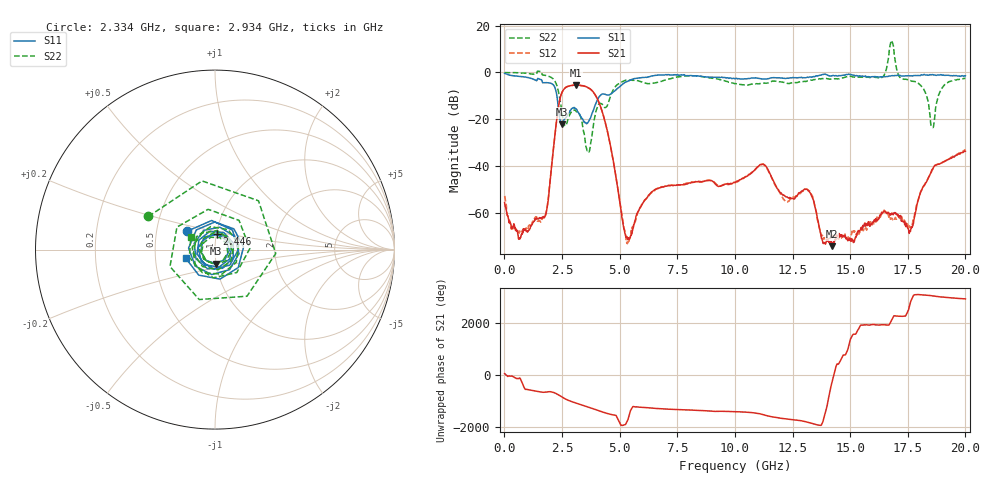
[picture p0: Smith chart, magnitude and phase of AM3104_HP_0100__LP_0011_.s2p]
!Created with skrf (http://scikit-rf.org).
# Hz S RI R 50.0
!freq ReS11 ImS11 ReS21 ImS21 ReS12 ImS12 ReS22 ImS22
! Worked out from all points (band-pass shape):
!   1601 points, 10 MHz to 20 GHz, reference 50 ohm
!   highest |S21| = -5.36 dB at 3.108 GHz (marker M1); lowest = -74.2 dB at 14.2 GHz (marker M2)
!   |S21| within 3 dB of the highest: 2.506 GHz to 3.857 GHz (1.351 GHz wide, 42.5 % of centre)
!   lowest |S11| = -22.2 dB at 2.496 GHz (marker M3), VSWR 1.17, Z = 49.7 - j7.77 ohm
!   |S11| at or under -10 dB: 2.279 GHz to 4.146 GHz (1.867 GHz wide, 58.1 % of centre)
!   |S22| runs from -34.0 to 13.7 dB; largest |S21 - S12| = 0.03
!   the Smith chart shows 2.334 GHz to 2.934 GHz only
!   S11 on the Smith chart (normalised r, x): 2.334 GHz: 0.72, +0.15; 2.446 GHz: 1.00, +0.17; 2.934 GHz: 0.72, -0.07
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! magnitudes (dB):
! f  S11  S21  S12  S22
! 10 MHz  -0.4  -55.6  -52.7  0.0
! 672.2 MHz  -1.7  -70.8  -67.7  -0.2
! 1.684 GHz  -4.4  -61.6  -62.0  -1.1
! 2.334 GHz  -14.7  -15.4  -15.5  -7.7
! 2.446 GHz  -21.3  -10.0  -10.0  -13.5
! 2.496 GHz  -22.2  -8.6  -8.6  -17.0
! 2.934 GHz  -15.4  -5.5  -5.6  -16.4
! 3.108 GHz  -15.6  -5.4  -5.4  -16.5
! 3.346 GHz  -19.4  -5.5  -5.6  -20.2
! 3.646 GHz  -21.1  -6.6  -6.7  -33.5
! 4.27 GHz  -9.2  -17.6  -17.6  -13.9
! 5.332 GHz  -3.8  -70.5  -73.1  -3.2
! 6.682 GHz  -1.1  -49.5  -49.3  -4.2
! 10.01 GHz  -2.7  -47.0  -47.0  -4.8
! 11.2 GHz  -2.8  -39.1  -39.3  -4.6
! 13.34 GHz  -2.0  -53.0  -52.4  -3.3
! 14.2 GHz  -1.5  -74.2  -70.6  -2.8
! 16.68 GHz  -1.5  -60.1  -61.8  7.2
! 17.63 GHz  -1.4  -67.2  -66.1  -3.5
! 18.56 GHz  -0.9  -41.3  -41.7  -23.4
! 19.01 GHz  -1.1  -38.4  -38.3  -6.3
! 20 GHz  -1.4  -33.7  -33.1  -2.5
